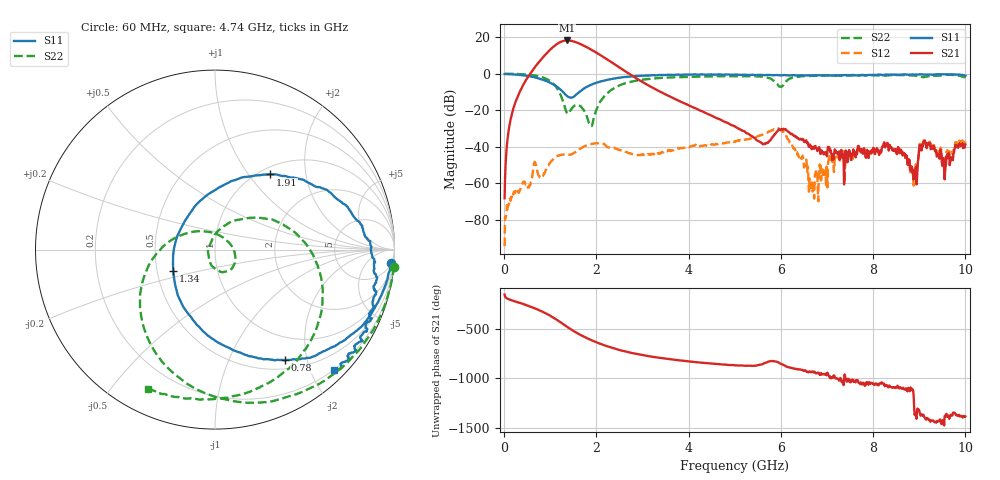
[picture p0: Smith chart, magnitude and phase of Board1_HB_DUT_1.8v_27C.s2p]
! Created Tue May 27 10:37:20 2025
# hz S ma R 50
! 2 Port Network Data from SP1.SP block
! freq  magS11  angS11  magS21  angS21  magS12  angS12  magS22  angS22
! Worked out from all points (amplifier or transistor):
!   1000 points, 10 MHz to 10 GHz, reference 50 ohm
!   highest |S21| = 18.3 dB at 1.36 GHz (marker M1)
!   |S21| within 3 dB of that: 1.089 GHz to 1.738 GHz (648.9 MHz wide, 45.9 % of centre)
!   unconditionally stable (mu >= 1): 58.04 MHz to 62.85 MHz; 88.48 MHz to 107.9 MHz; 112.7 MHz to end of sweep
!   at 1.67 GHz: K = 7.38, MAG = 16.7 dB, |S12| = -40.7 dB
!   at 5.01 GHz: K = 18.12, MAG = -11.6 dB, |S12| = -37.0 dB
!   at 10 GHz: K = 220.06, MAG = -27.3 dB, |S12| = -37.1 dB
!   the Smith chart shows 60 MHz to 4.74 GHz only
!   S11 on the Smith chart (normalised r, x): 60 MHz: 6, -25; 780 MHz: 0.62, -1.63; 1.34 GHz: 0.61, -0.16; 1.91 GHz: 1.11, +1.27; 4.74 GHz: 0.19, -2.39
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1e7  0.981 -1.0  0.0003924 -152.2  1.92e-05 -41.8  1.005 -0.8
6e7  0.9831 -4.3  0.01132 168.5  0.0002559 95.8  0.9992 -5.5
5.1e8  0.8745 -35.9  0.7984 95.9  0.0007769 90.7  0.9517 -50.2
7.8e8  0.7283 -57.8  2.301 45.0  0.001418 81.7  0.8387 -85.5
9.5e8  0.6083 -74.2  3.977 6.0  0.003058 117.1  0.6913 -115.2
1.11e9  0.4783 -95.2  6.09 -37.6  0.00522 99.6  0.4655 -152.2
1.24e9  0.3544 -121.4  7.608 -78.2  0.006043 82.5  0.2356 164.7
1.34e9  0.2627 -152.7  8.158 -110.6  0.006043 75.0  0.09735 100.9
1.36e9  0.2476 -160.9  8.186 -117.0  0.006001 74.5  0.0853 80.2
1.51e9  0.2361 131.2  7.664 -162.3  0.006755 77.1  0.1288 -30.2
1.68e9  0.3555 83.8  6.292 153.2  0.009473 69.2  0.1203 -79.7
1.91e9  0.5183 53.9  4.424 102.5  0.01214 44.8  0.04005 129.5
2.27e9  0.7005 28.6  2.314 39.1  0.009637 9.5  0.3189 33.0
2.66e9  0.8289 9.3  1.099 -12.0  0.007212 -2.4  0.5685 -7.0
3.34e9  0.9181 -14.4  0.345 -70.3  0.006737 11.5  0.763 -52.2
4.74e9  0.9443 -45.2  0.05143 -140.0  0.01245 -4.1  0.8605 -115.8
5.01e9  0.9615 -50.3  0.03576 -148.5  0.01415 -10.4  0.8642 -126.3
5.98e9  0.9095 -70.1  0.0295 -128.7  0.02926 -99.9  0.4485 -152.7
6.67e9  0.9052 -90.6  0.008598 148.1  0.001061 -56.9  0.8871 -156.3
8.34e9  0.9397 -136.7  0.007925 -4.9  0.008298 -10.7  0.9069 167.2
8.9e9  0.9514 -147.5  0.001667 70.7  0.00251 66.6  0.8961 155.0
1e10  0.8865 -164.9  0.01153 55.3  0.01404 55.1  0.8173 137.9
